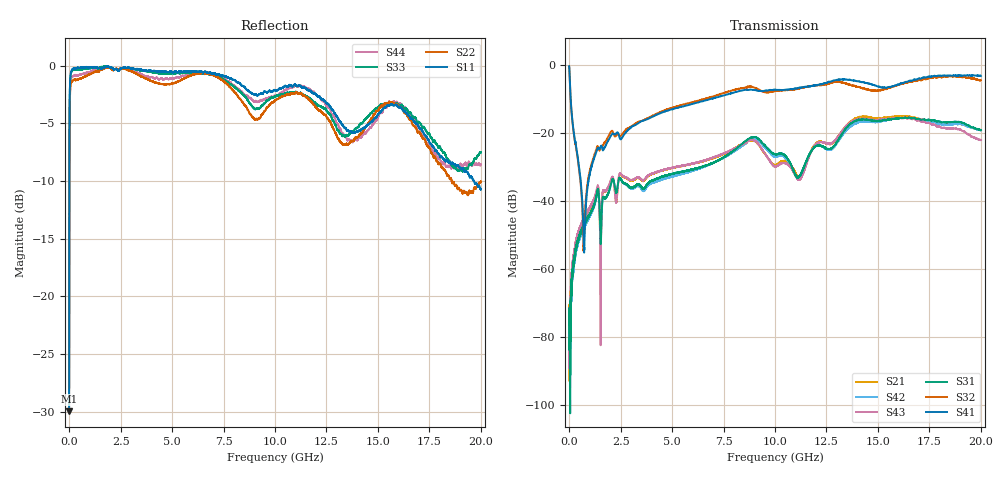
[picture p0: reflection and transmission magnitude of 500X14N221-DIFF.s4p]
! Created Wed Oct 27 15:54:01 2021
# hz S ma R 50
! 4 Port Network Data from SP1.SP block
! freq  magS11  angS11  magS12  angS12  magS13  angS13  magS14  angS14
!  magS21  angS21  magS22  angS22  magS23  angS23  magS24  angS24
!  magS31  angS31  magS32  angS32  magS33  angS33  magS34  angS34
!  magS41  angS41  magS42  angS42  magS43  angS43  magS44  angS44
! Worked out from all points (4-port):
!   20001 points, 300 kHz to 20 GHz, reference 50 ohm
!   strongest paths, dB at 300 kHz, 5 GHz, 10 GHz, 15 GHz, 20 GHz:
!     S41: -0.3, -13.0, -7.2, -6.3, -3.1
!     S32: -0.4, -12.5, -7.6, -7.5, -4.4
!     S31: -81.7, -32.0, -26.2, -16.4, -19.1
!     S43: -84.1, -30.2, -29.8, -16.1, -22.0
!     S42: -83.9, -32.8, -26.9, -16.7, -19.2
!     S21: -92.9, -30.3, -29.4, -15.7, -19.1
!   lowest |S11| = -30.0 dB at 300 kHz (marker M1), VSWR 1.07, Z = 53 - j1.37 ohm
!   |S11| at or under -10 dB: start of sweep to 9.098 MHz; 19.67 GHz to end of sweep
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300000  0.03172 -24.1  1.104e-05 -61.1  0.0001186 -84.5  0.9686 -0.7
        2.266e-05 79.5  0.04002 -16.4  0.9581 -0.6  0.0001381 69.8
        8.245e-05 123.6  0.9604 -0.5  0.04016 -17.8  0.0001452 -67.8
        0.9697 -0.7  6.365e-05 100.3  6.236e-05 -89.1  0.03111 -22.0
1.203e8  0.9538 -168.6  0.0007 103.7  0.0006209 107.9  0.2064 -78.2
         0.0007533 101.9  0.8542 -168.6  0.1989 -78.2  0.0005335 110.4
         0.0006109 108.1  0.1989 -78.3  0.9453 -168.5  0.000695 99.9
         0.2058 -78.3  0.0005212 108.0  0.0007588 101.9  0.8916 -168.5
7.353e8  0.9804 174.3  0.005463 82.7  0.004513 80.9  0.001887 15.2
         0.005606 82.2  0.8962 172.4  0.003336 50.1  0.004212 80.7
         0.004507 80.7  0.003386 50.1  0.97 173.1  0.005625 81.2
         0.001902 13.0  0.004129 82.2  0.005703 81.4  0.9258 172.4
1.3383e9  0.9828 167.8  0.01416 62.6  0.01245 57.3  0.05521 72.8
          0.01414 62.4  0.9469 165.9  0.05999 71.0  0.01198 59.5
          0.01237 56.6  0.06024 71.1  0.9829 166.2  0.01471 61.6
          0.05494 72.8  0.01188 59.5  0.01468 61.2  0.9644 166.0
4.7763e9  0.9392 145.5  0.02957 44.7  0.02415 36.8  0.2145 55.4
          0.02961 45.0  0.8329 146.4  0.2242 55.3  0.022 37.9
          0.024 36.4  0.2247 55.4  0.9266 146.2  0.02991 45.7
          0.2137 55.3  0.02222 37.6  0.02993 45.3  0.8788 147.5
1.41053e10  0.5224 80.1  0.1744 17.3  0.1575 16.3  0.5775 -33.8
            0.174 17.6  0.502 96.0  0.4742 -36.8  0.1466 20.2
            0.1584 16.7  0.477 -36.7  0.5543 97.7  0.1643 20.7
            0.5766 -33.5  0.1465 20.4  0.1626 20.9  0.4939 85.0
2e10  0.2904 45.6  0.1102 157.1  0.11 162.4  0.6993 -79.4
      0.1106 156.9  0.3155 65.0  0.6034 -83.8  0.1106 165.2
      0.1108 162.8  0.6027 -83.2  0.4205 72.3  0.07985 167.5
      0.6985 -79.2  0.1099 165.6  0.07927 167.4  0.3747 56.5
